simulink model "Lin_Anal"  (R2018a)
settings: Solver=ode4  StartTime=0.0  StopTime=1  FixedStep=Ts  MaxStep=0.5  RelTol=1e-3  EnableMultiTasking=on
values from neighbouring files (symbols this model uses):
  ini = [wb0; atto; Hco]    [run.m]
  Kq1 = I22*ww^2 - 3*wo2*(I11-I33)    [run.m]
  Kq2 = 2*I22*zet*ww    [run.m]
  Kqi = 0.0005    [run.m]
  Kr1 = (0.1*I11*I33*zet^2/Hy0) - sqrt( ((0.01^zet^4*I11^2*I33^2)/Hy0^2)+(4*I11*I33*zet^2) )    [run.m]
  Kr2 = 0.05*Kr1    [run.m]
  Kr3 = 0.04*zet*(Kr2-Hy0) * sqrt(abs(Hy0/(I11*I33)))    [run.m]
  nt = 7    [run.m]    (also in runf.m)
  Ts = 0.001    [run.m]    (also in runf.m = 0.0005)
undefined symbols (not defined in the file or in its folder): DiscIntNeverNeededParam, NonLin_Vehi_Dynamics, RW_Steering
libraries: simulink x3

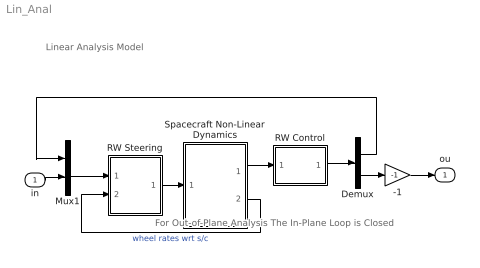
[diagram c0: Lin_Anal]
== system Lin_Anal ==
  note: Linear Analysis Model
  note: For Out-of-Plane Analysis The In-Plane Loop is Closed
  in : Inport
  -1 : Gain  Gain=-1
  Demux : Demux  Outputs=2
  Mux1 : Mux  Inputs=2
  RW Control : Subsystem
  RW Steering : Subsystem
  Spacecraft Non-Linear Dynamics : Subsystem
  ou : Outport
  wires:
  Spacecraft Non-Linear Dynamics/1(att-lv) -> RW Control/1(atti)
  RW Control/1(Tc) -> Demux/1
  RW Steering/1(Twi) -> Spacecraft Non-Linear Dynamics/1(Twi)
  Spacecraft Non-Linear Dynamics/2(wr) -> RW Steering/2(wr(1))  "wheel rates wrt s/c"
  Mux1/1 -> RW Steering/1(Trwc)
  -1/1 -> ou/1
  in/1 -> Mux1/2
  Demux/2 -> -1/1
  Demux/1 -> Mux1/1

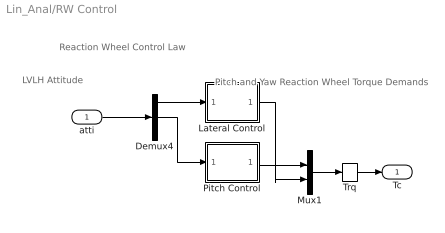
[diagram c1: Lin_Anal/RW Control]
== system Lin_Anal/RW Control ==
  note: Reaction Wheel Control Law
  note: LVLH Attitude
  note: Pitch and Yaw Reaction Wheel Torque Demands
  atti : Inport
  Demux4 : Demux  Outputs=3
  Lateral Control : Subsystem
  Mux1 : Mux  Inputs=2
  Pitch Control : Subsystem
  Trq : Memory
  Tc : Outport
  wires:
  Trq/1 -> Tc/1
  Lateral Control/1(Tcz) -> Mux1/2
  atti/1 -> Demux4/1
  Mux1/1 -> Trq/1
  Demux4/2 -> Pitch Control/1(the)
  Pitch Control/1(Tcy) -> Mux1/1
  Demux4/1 -> Lateral Control/1(phi)

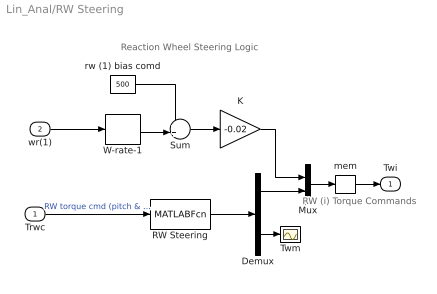
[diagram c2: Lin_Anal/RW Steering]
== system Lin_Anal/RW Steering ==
  note: Reaction Wheel Steering Logic
  note: RW (i) Torque Commands
  Trwc : Inport
  wr(1) : Inport  Port=2
  Demux : Demux  Outputs=[2, 1]
  K : Gain  Gain=-0.02
  Mux : Mux  Inputs=[1,2]
  RW Steering : MATLABFcn  MATLABFcn=RW_Steering( u(1:2) )  OutputDimensions=3
  Sum : Sum  Inputs=++|
  Twm : Scope
  W-rate-1 : Selector  InputPortWidth=3  IndexOptions=Index vector (dialog)  Indices=[1]  OutputSizes=1
  mem : Memory
  rw (1) bias comd : Constant  Value=500
  Twi : Outport
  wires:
  mem/1 -> Twi/1
  K/1 -> Mux/1
  W-rate-1/1 -> Sum/2
  rw (1) bias comd/1 -> Sum/1
  Sum/1 -> K/1
  wr(1)/1 -> W-rate-1/1
  Mux/1 -> mem/1
  Trwc/1 -> RW Steering/1  "RW torque cmd (pitch & yaw)"
  RW Steering/1 -> Demux/1
  Demux/1 -> Mux/2
  Demux/2 -> Twm/1

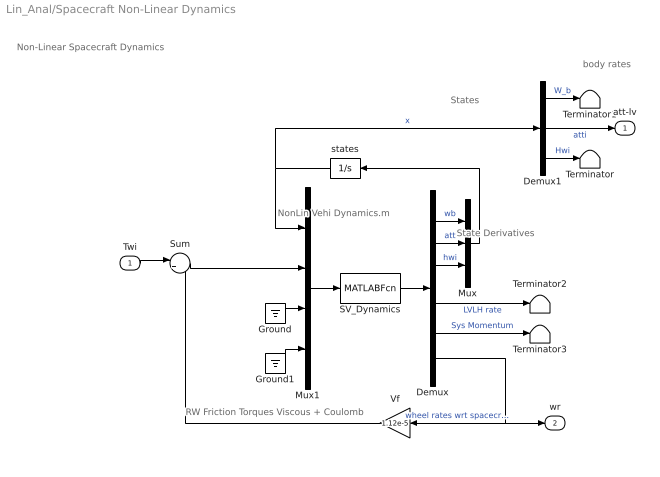
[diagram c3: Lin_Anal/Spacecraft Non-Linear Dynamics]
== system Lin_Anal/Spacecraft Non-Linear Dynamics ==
  note: State Derivatives
  note: body rates
  note: States
  note: RW Friction Torques Viscous + Coulomb
  note: Non-Linear Spacecraft Dynamics
  note: NonLin Vehi Dynamics.m
  Twi : Inport
  Demux : Demux  Outputs="[3,3,3,  3,3,3]"
  Demux1 : Demux  Outputs=[3,3,3]
  Ground : Ground
  Ground1 : Ground
  Mux : Mux  Inputs=[3,3,3]
  Mux1 : Mux  Inputs=[9,3, nt, 3]
  SV_Dynamics : MATLABFcn  MATLABFcn=NonLin_Vehi_Dynamics( u(1:9), u(10:12), u(13:12+nt), u(13+nt:15+nt) )  OutputDimensions=9+9
  Sum : Sum  Inputs=|+-
  Terminator{,1..3} (4 alike) : Terminator
  Vf : Gain  Gain=1.12e-5
  states : Integrator  InitialCondition=ini
  att-lv : Outport
  wr : Outport  Port=2
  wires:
  Demux/6 -> wr/1, Vf/1  "wheel rates wrt spacecrft"
  Demux1/2 -> att-lv/1  "atti"
  Mux1/1 -> SV_Dynamics/1
  SV_Dynamics/1 -> Demux/1
  states/1 -> Demux1/1, Mux1/1  "x"
  Vf/1 -> Sum/2
  Twi/1 -> Sum/1
  Sum/1 -> Mux1/2
  Ground/1 -> Mux1/3
  Demux/1 -> Mux/1  "wb"
  Demux/2 -> Mux/2  "att"
  Demux/3 -> Mux/3  "hwi"
  Mux/1 -> states/1
  Demux1/3 -> Terminator/1  "Hwi"
  Demux1/1 -> Terminator1/1  "W_b"
  Demux/4 -> Terminator2/1  "LVLH rate"
  Demux/5 -> Terminator3/1  "Sys Momentum"
  Ground1/1 -> Mux1/4

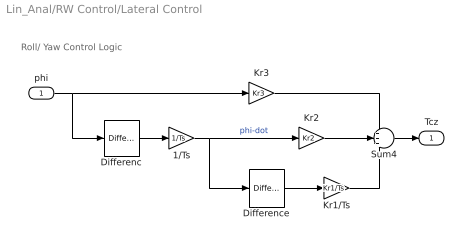
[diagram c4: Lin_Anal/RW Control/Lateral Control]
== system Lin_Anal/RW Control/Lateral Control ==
  note: Roll/ Yaw Control Logic
  phi : Inport
  1/Ts : Gain  Gain=1/Ts
  Differenc : simulink/Discrete/Difference  ICPrevInput=0.0  InputProcessing=Inherited  OutMin=[]  OutMax=[]  OutDataType=sfix(16)  OutScaling=2^-10  DoSatur=off
  Difference : simulink/Discrete/Difference  ICPrevInput=0.0  InputProcessing=Inherited  OutMin=[]  OutMax=[]  OutDataType=sfix(16)  OutScaling=2^-10  DoSatur=off
  Kr1/Ts : Gain  Gain=Kr1/Ts
  Kr2 : Gain  Gain=Kr2
  Kr3 : Gain  Gain=Kr3
  Sum4 : Sum  Inputs=+++
  Tcz : Outport
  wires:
  1/Ts/1 -> Difference/1, Kr2/1  "phi-dot"
  Differenc/1 -> 1/Ts/1
  Difference/1 -> Kr1/Ts/1
  Sum4/1 -> Tcz/1
  phi/1 -> Differenc/1, Kr3/1
  Kr1/Ts/1 -> Sum4/3
  Kr2/1 -> Sum4/2
  Kr3/1 -> Sum4/1

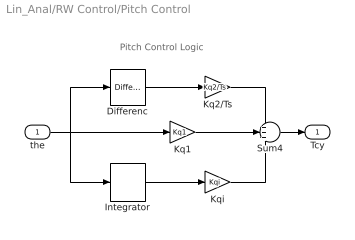
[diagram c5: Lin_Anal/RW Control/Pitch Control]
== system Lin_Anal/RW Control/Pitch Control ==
  note: Pitch Control Logic
  the : Inport
  Differenc : simulink/Discrete/Difference  ICPrevInput=0.0  InputProcessing=Inherited  OutMin=[]  OutMax=[]  OutDataType=sfix(16)  OutScaling=2^-10  DoSatur=off
  Integrator : DiscreteIntegrator  SampleTime=Ts  ICPrevOutput=DiscIntNeverNeededParam  ICPrevScaledInput=DiscIntNeverNeededParam
  Kq1 : Gain  Gain=Kq1
  Kq2/Ts : Gain  Gain=Kq2/Ts
  Kqi : Gain  Gain=Kqi
  Sum4 : Sum  Inputs=+++
  Tcy : Outport
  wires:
  Differenc/1 -> Kq2/Ts/1
  Integrator/1 -> Kqi/1
  Kqi/1 -> Sum4/3
  the/1 -> Differenc/1, Integrator/1, Kq1/1
  Kq2/Ts/1 -> Sum4/1
  Sum4/1 -> Tcy/1
  Kq1/1 -> Sum4/2
